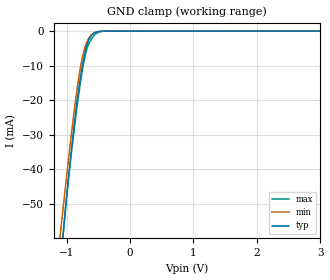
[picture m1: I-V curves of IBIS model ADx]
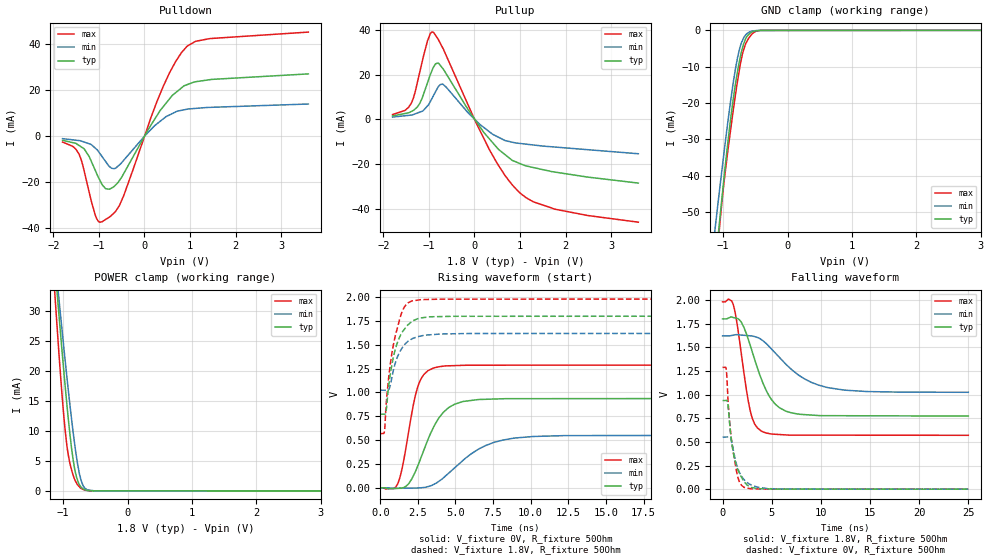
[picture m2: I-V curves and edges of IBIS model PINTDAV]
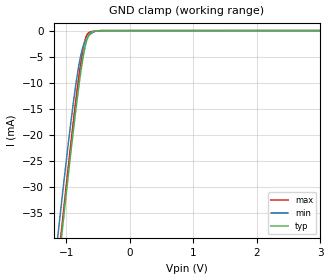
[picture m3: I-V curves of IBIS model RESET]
|Texas Instruments Incorporated
|12-Bit, Nanopower, 4-Wire TOUCH SCREEN CONTROLLER with I2C Interface
| Marketing part#   Digital Voltage Range   Package-type   #pins
| TSC2013QRSARQ1   1.6V to 3.6V   QFN   16
| TSC2013QPWRQ1   1.6V to 3.6V   TSSOP   16
[IBIS Ver]   4.0
[File name]   tsc2013-q1.ibs
[File Rev]   1.0
[Date]   04/07/2014
[Source]
| Texas Instruments Incorporated.
| Analog-eLab, HPA
| 12500 TI Blvd
| Dallas, TX -75243
[Notes]   Revision History:
| Rev 1.0: 04/07/2014
| - Initial version of the model
| - Initial Model generated from simulations in TISPICED
| - Model names contains the model for 1.8V(1.62V and 1.98V, +/- 10%).
| - Model not matched to measurements
| - Ignore warnings related to min and max values of ccomp,
|   The device process of these products is CMOS. The ccomp
|   values are based on PVT variations as seen in simulations
| - tsc2013.ibs model is used to create Package IBIS model for TSC2013-Q1.
[Disclaimer]
| This product is designed as an aid for customers of Texas Instruments.
| No warranties, either expressed or implied, with respect to this third
| party software (if any) or with respect to its fitness for any
| particular purpose is claimed by Texas Instruments or the author. The
| software (if any) is provided solely on an "as is" basis. The entire
| risk as to its quality and performance is with the customer
[Copyright]
(C) Copyright 2010 Texas Instruments Incorporated.All rights reserved.
|   TSC2013-Q1RSA
[Component]   TSC2013-Q1RSA
[Manufacturer]   TI
[Package]   |16 QFN  -  RSA package
|   typ   min   max
R_pkg   0.06676   0.06329   0.06959
L_pkg   1.12902nH   1.0598nH   1.18576nH
C_pkg   0.163855pF   0.16006pF   0.17031pF
[Pin]  signal_name   model_name   R_pin   L_pin   C_pin
1   SDA   SDA   0.06701   1.13606nH   0.16006pF
2   SCL   SCL   0.06329   1.0598nH   0.16988pF
3   AD1   ADx   0.06532   1.0985nH   0.17031pF
4   _PINTDAV   PINTDAV   0.06959   1.18576nH   0.16091pF
5   _RESET   RESET   0.06682   1.13036nH   0.16126pF
6   DGND   GND   0.03183   0.73349nH   0.2072pF
7   I/OVDD   POWER   0.03431   0.81566nH   0.21459pF
8   AUX   NC   0.08038   1.38887nH   0.17667pF
9   AGND   GND   0.03096   0.82932nH   0.18257pF
10   SNSVDD/VREF   POWER   0.02125   0.57292nH   0.24326pF
11   X+   NC   0.0322   0.7431nH   0.20583pF
12   Y+   NC   0.03399   0.80877nH   0.19302pF
13   X-   NC   0.03324   0.79109nH   0.19012pF
14   Y-   NC   0.03226   0.75057nH   0.20698pF
15   SNSGND   GND   0.03242   0.75308nH   0.20701pF
16   AD0   ADx   0.06853   1.16366nH   0.16071pF
|   TSC2013-Q1PW
[Component]   TSC2013-Q1PW
[Manufacturer]   TI
[Package]   |16 TSSOP  -  PW package
|   typ   min   max
R_pkg   0.0695416   0.06275   0.07818
L_pkg   2.359185nH   2.01178nH   2.98235nH
C_pkg   0.4143116pF  0.37102pF   0.50201pF
[Pin]  signal_name   model_name   R_pin   L_pin   C_pin
1   AD0   ADx   0.06643   2.98235nH   0.48546pF
2   SDA   SDA   0.07818   2.69435nH   0.50201pF
3   SCL   SCL   0.06987   2.15384nH   0.37309pF
4   AD1   ADx   0.06545   2.06324nH   0.37377pF
5   _PINTDAV   PINTDAV   0.06275   2.01178nH   0.37102pF
6   _RESET   RESET   0.07457   2.24955nH   0.38052pF
7   DGND   GND   0.04246   2.40576nH   0.54792pF
8   I/OVDD   POWER   0.03949   2.82552nH   0.52699pF
9   AUX   NC   0.07434   3.14354nH   0.49417pF
10   AGND   GND   0.03565   2.16942nH   0.52387pF
11   SNSVDD/VREF   POWER   0.02594   1.70027nH   0.45323pF
12   X+   NC   0.03552   1.81582nH   0.41431pF
13   Y+   NC   0.03349   1.74161nH   0.40619pF
14   X-   NC   0.03804   1.91217nH   0.4075pF
15   Y-   NC   0.04807   2.60792nH   0.56692pF
16   SNSGND   GND   0.04281   2.94689nH   0.53819pF
| Models and submodels in the file (5): ADx (Input), PINTDAV (3-state), RESET (Input), SCL (Input), SDA (I/O_open_drain)
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|   1.8V ADx Model
[Model] ADx
Model_type Input
Vinl = 0.54
Vinh = 1.26
|   typ   min   max
|   (nom PVT)   (Fast PVT)   (Slow PVT)
C_comp   8.27255E-12  7.84431E-12   8.94629E-12
|Where nom PVT is NOM Process, 1.8V,27C
|   Fast PVT is Strong Process, 2.07V, -40C
|   Slow PVT is Weak Process, 1.53V, 85C
[Voltage Range]   1.8   1.62   1.98
[Temperature Range]   30   88   -40
[Power Clamp Reference]   1.8   1.62   1.98
[GND Clamp Reference]   0   0   0
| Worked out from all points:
|   GND clamp passes 1 mA (typ) near -0.59 V on its own axis
[GND Clamp]
|   Voltage   I(typ)   I(min)   I(max)
-1.8V     -218.2mA   -187.6mA   -259.9mA
-1.098V   -68.02mA   -59.02mA   -69.19mA
-1.058V   -60.05mA   -52.15mA   -59.93mA
-1.036V   -55.66mA   -48.36mA   -55.33mA
-977.3mV  -44.33mA   -38.53mA   -44.08mA
-909.6mV  -32.25mA   -27.73mA   -33.18mA
-787.9mV  -14.33mA   -11.26mA   -15.82mA
-731.4mV  -8.267mA   -6.111mA   -9.335mA
-680.7mV  -4.196mA   -3.295mA   -5.229mA
-570.9mV  -694.3uA   -529.4uA   -1.435mA
-418.2mV  -20.93uA   -22.61uA   -27.08uA
3.6V      0A         0A         0A
[POWER Clamp]
|   SCR cell for ESD function. Effects occurr above VDD x 2
|   Voltage   I(typ)   I(min)   I(max)
-1.8V     0A         0A         0A
0V        0A         0A         0A
3.6V      0A         0A         0A
|   1.8V PINTDAV Model
[Model] PINTDAV
Model_type 3-state
Polarity   Non-Inverting
Enable   Active-Low
Vmeas = 0.9
Vref = 0.9
Cref = 15pF
Rref = 50
|   typ   min   max
|   (Fast PVT)   (nom PVT)   (Slow PVT)
|   C_comp high impedance
C_comp   8.58302E-12   8.34919E-12   8.86424E-12
|   C_comp high output
|C_comp   9.19686E-12   9.07071E-12   9.36789E-12
|   C_comp low output
|C_comp   9.11254E-12   8.94629E-12   9.15466E-12
|Where nom PVT is NOM Process, 1.8V,27C
|   Fast PVT is Strong Process, 2.07V, -40C
|   Slow PVT is Weak Process, 1.53V, 85C
[Voltage Range]   1.8   1.62   1.98
[Temperature Range]   30   88   -40
[Pullup Reference]   1.8   1.62   1.98
[Pulldown Reference]   0   0   0
[Power Clamp Reference]   1.8   1.62   1.98
[GND Clamp Reference]   0   0   0
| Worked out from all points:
|   slope of the pulldown table from 0 to 0.27 V, typ, clamps not added: 30.6 ohm
|   slope of the pullup table from 0 to 0.27 V, typ, clamps not added: 35.6 ohm
|   GND clamp passes 1 mA (typ) near -0.60 V on its own axis
|   POWER clamp passes 1 mA (typ) near -0.75 V on its own axis
|   falling waveform, V_fixture 1.8V, R_fixture 50Ohm: 20-80 % time 2.21ns typ, 3.96ns min, 1.22ns max; typ from 1.8 V to 0.773 V
|   rising waveform, V_fixture 0V, R_fixture 50Ohm: 20-80 % time 1.59ns typ, 2.73ns min, 917ps max; typ from 0 V to 0.936 V
|   rising waveform, V_fixture 1.8V, R_fixture 50Ohm: 20-80 % time 831ps typ, 847ps min, 793ps max; typ from 0.773 V to 1.8 V
|   falling waveform, V_fixture 0V, R_fixture 50Ohm: 20-80 % time 953ps typ, 1.06ns min, 795ps max; typ from 0.936 V to 0 V
[Pulldown]
|   Voltage   I(typ)   I(min)   I(max)
-1.8V     -1.785mA   -1.085mA   -2.549mA
-1.44V    -3.998mA   -1.903mA   -7.738mA
-1.323V   -5.565mA   -2.57mA    -15.26mA
-1.086V   -14.65mA   -5.123mA   -33.99mA
-936.4mV  -20.79mA   -8.718mA   -37.14mA
-723.9mV  -22.51mA   -13.9mA    -34.3mA
-552.1mV  -19.24mA   -12.48mA   -30.13mA
407.3mV   12.67mA    7.427mA    21.39mA
685.6mV   18.88mA    10.52mA    32.4mA
932.2mV   22.31mA    11.67mA    38.92mA
1.439V    24.5mA     12.48mA    42.32mA
3.6V      27mA       13.94mA    45.13mA
[GND Clamp]
|   Voltage   I(typ)   I(min)   I(max)
-1.8V     -195.6mA   -164.2mA   -238.9mA
-1.116V   -63.55mA   -53.15mA   -66.95mA
-1.06V    -53.49mA   -44.64mA   -55.05mA
-1.044V   -50.54mA   -42.14mA   -51.93mA
-1.003V   -43.37mA   -36.03mA   -44.42mA
-924.7mV  -30.49mA   -24.89mA   -32.82mA
-804.8mV  -14.27mA   -10.19mA   -17.3mA
-743.3mV  -8.187mA   -5.003mA   -10.37mA
-697.2mV  -4.668mA   -2.688mA   -6.288mA
-592.4mV  -958.7uA   -452uA     -1.892mA
-418.1mV  -20.23uA   -20.33uA   -27.04uA
3.6V      0A         0A         0A
[Pullup]
|   Voltage   I(typ)   I(min)   I(max)
-1.8V     1.553mA    1.028mA    2.153mA
-1.385V   3.554mA    1.925mA    7.371mA
-1.201V   7.19mA     3.233mA    21.22mA
-1.033V   16.39mA    6.01mA     35.09mA
-915.6mV  22.78mA    10.07mA    39.05mA
-804.8mV  25.21mA    14.29mA    36.06mA
-689.5mV  22.56mA    15.62mA    31.64mA
324.9mV   -8.666mA   -5.516mA   -13.45mA
667.4mV   -15.71mA   -9.438mA   -25.01mA
983.6mV   -19.64mA   -10.74mA   -32.64mA
1.766V    -23.58mA   -12.38mA   -40.16mA
3.6V      -28.5mA    -15.38mA   -46mA
[POWER Clamp]
|   Voltage   I(typ)   I(min)   I(max)
-1.8V     130.3mA    116.1mA    148.7mA
-1.146V   39.82mA    40.79mA    35.57mA
-1.124V   36.87mA    38.27mA    31.92mA
-1.084V   31.72mA    33.96mA    25.76mA
-1.066V   29.45mA    32.01mA    22.99mA
-996.5mV  20.74mA    24.56mA    13.25mA
-936.4mV  13.75mA    18.39mA    7.103mA
-818.9mV  3.531mA    7.618mA    1.856mA
-726.8mV  715uA      1.969mA    446.5uA
-655.8mV  182.2uA    387.2uA    114.6uA
-510.9mV  11.18uA    9.084uA    15.41uA
3.6V      0A         0A         0A
[Ramp]
R_load = 50
|   typ   min   max
dV/dt_r   0.561804/1.5861e-009   0.329858/2.71124e-009  0.772232/9.12939e-010
dV/dt_f   0.616387/2.19461e-009  0.357543/3.92282e-009  0.846341/1.21582e-009
[Falling Waveform]
V_fixture = 1.8V
V_fixture_min = 1.62V
V_fixture_max = 1.98V
R_fixture = 50Ohm
|   Time   V(typ)   V(min)   V(max)
0s        1.8V       1.62V      1.98V
1.101ns   1.815V     1.628V     1.946V
1.913ns   1.764V     1.629V     1.427V
2.787ns   1.529V     1.621V     841.8mV
3.258ns   1.374V     1.613V     690.4mV
3.967ns   1.159V     1.58V      612.9mV
5.791ns   860.6mV    1.392V     577.5mV
8.3ns     788.4mV    1.168V     571.2mV
10.56ns   777mV      1.077V     570.9mV
25ns      772.7mV    1.024V     569.4mV
[Rising Waveform]
V_fixture = 0V
V_fixture_min = 0V
V_fixture_max = 0V
R_fixture = 50Ohm
|   Time   V(typ)   V(min)   V(max)
0s        1.186nV    132.3nV    24.56nV
1.157ns   -5.895mV   -5.949mV   40.9mV
1.829ns   32.25mV    -4.006mV   534.1mV
2.464ns   218.5mV    -2.169mV   1.044V
2.883ns   389.1mV    2.598mV    1.185V
3.529ns   631.6mV    33.06mV    1.256V
4.929ns   875.7mV    206.9mV    1.282V
6.591ns   926.2mV    410.5mV    1.286V
8.785ns   934.8mV    518.3mV    1.286V
25ns      936.3mV    549.8mV    1.287V
[Rising Waveform]
V_fixture = 1.8V
V_fixture_min = 1.62V
V_fixture_max = 1.98V
R_fixture = 50Ohm
|   Time   V(typ)   V(min)   V(max)
0s        772.7mV    1.024V     569.4mV
281.2ps   771.7mV    1.023V     593.1mV
395.9ps   812mV      1.022V     885mV
564.4ps   1.074V     1.031V     1.164V
760.9ps   1.282V     1.147V     1.4V
982.4ps   1.442V     1.298V     1.583V
1.503ns   1.643V     1.479V     1.867V
2.065ns   1.739V     1.559V     1.958V
4.899ns   1.799V     1.616V     1.979V
25ns      1.8V       1.62V      1.98V
[Falling Waveform]
V_fixture = 0V
V_fixture_min = 0V
V_fixture_max = 0V
R_fixture = 50Ohm
|   Time   V(typ)   V(min)   V(max)
0s        936.3mV    549.8mV    1.287V
376.9ps   937.9mV    551.2mV    1.264V
547.9ps   889.4mV    551.9mV    956.6mV
780ps     626.8mV    545.4mV    638.4mV
1.063ns   404.8mV    431.3mV    409.8mV
1.386ns   258.6mV    275.4mV    209.9mV
1.716ns   167mV      177.2mV    77.02mV
2.187ns   78.49mV    100.7mV    19.29mV
4.711ns   2.222mV    5.364mV    775.9uV
25ns      1.779nV    132.4nV    10.96nV
|   1.8V RESET Model
[Model] RESET
Model_type Input
Vinl = 0.54
Vinh = 1.26
|   typ   min   max
|   (nom PVT)   (Fast PVT)   (Slow PVT)
C_comp   7.9367E-12   7.75609E-12   8.23458E-12
|Where nom PVT is NOM Process, 1.8V,27C
|   Fast PVT is Strong Process, 2.07V, -40C
|   Slow PVT is Weak Process, 1.53V, 85C
[Voltage Range]   1.8   1.62   1.98
[Temperature Range]   30   88   -40
[Power Clamp Reference]   1.8   1.62   1.98
[GND Clamp Reference]   0   0   0
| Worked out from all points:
|   GND clamp passes 1 mA (typ) near -0.65 V on its own axis
[GND Clamp]
|   Voltage   I(typ)   I(min)   I(max)
-1.8V     -125.7mA   -117.6mA   -125.2mA
-1.122V   -45.13mA   -38.33mA   -43.79mA
-1.076V   -39.84mA   -33.26mA   -38.44mA
-1.049V   -36.81mA   -30.3mA    -35.36mA
-924.8mV  -23.06mA   -17.35mA   -21.37mA
-812mV    -11.61mA   -7.408mA   -9.741mA
-753.3mV  -6.496mA   -3.847mA   -4.758mA
-721.7mV  -4.233mA   -2.605mA   -2.666mA
-676.7mV  -1.855mA   -1.471mA   -880.1uA
-646.4mV  -903.8uA   -987.7uA   -402.4uA
-459.2mV  -7.729uA   -14.08uA   -22.74uA
3.6V      0A         0A         0A
[POWER Clamp]
|   SCR cell for ESD function. Effects occurr above VDD x 2
|   Voltage   I(typ)   I(min)   I(max)
-1.8V     0A         0A         0A
0V        0A         0A         0A
3.6V      0A         0A         0A
